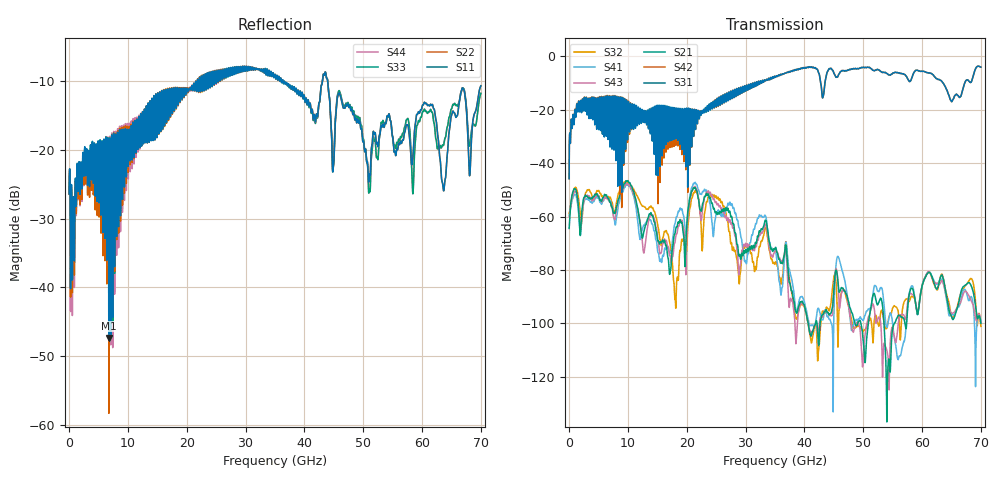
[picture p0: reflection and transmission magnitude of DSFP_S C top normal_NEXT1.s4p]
! AWR Design Environment (8415) Wed Jan 09 11:05:57 2019
! Document = 'DSFP_S'
! nPorts: 4, nXvals: 7001
# HZ S DB R 50
!Freq DBS11 AngS11 DBS12 AngS12 DBS13 AngS13 DBS14 AngS14
!	DBS21 AngS21 DBS22 AngS22 DBS23 AngS23 DBS24 AngS24
!	DBS31 AngS31 DBS32 AngS32 DBS33 AngS33 DBS34 AngS34
!	DBS41 AngS41 DBS42 AngS42 DBS43 AngS43 DBS44 AngS44
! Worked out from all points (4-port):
!   7000 points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, 10 MHz to 70 GHz, reference 50 ohm
!   strongest paths, dB at 10 MHz, 17.51 GHz, 35.01 GHz, 52.51 GHz, 70 GHz:
!     S31: -45.8, -27.6, -7.6, -5.0, -4.0
!     S42: -45.8, -28.8, -7.6, -5.0, -4.0
!     S21: -64.4, -73.0, -72.0, -92.8, -99.9
!     S43: -60.1, -75.6, -73.0, -98.2, -99.8
!     S41: -59.4, -69.8, -72.9, -87.9, -98.9
!     S32: -58.8, -75.9, -77.8, -100.1, -101.1
!   lowest |S11| = -47.4 dB at 6.75 GHz (marker M1), VSWR 1.01, Z = 49.8 + j0.367 ohm
!   |S11| at or under -10 dB: start of sweep to 21.81 GHz; 36.37 GHz to 43.07 GHz (6.701 GHz wide, 16.9 % of centre); 43.96 GHz to end of sweep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
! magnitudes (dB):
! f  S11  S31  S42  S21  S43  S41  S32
! 10 MHz  -26.4  -45.8  -45.8  -64.4  -60.1  -59.4  -58.8
! 1.63 GHz  -23.0  -16.8  -16.7  -57.6  -56.7  -59.0  -53.5
! 6.75 GHz  -47.4  -16.0  -15.8  -53.6  -53.8  -53.4  -52.6
! 17.98 GHz  -12.1  -19.2  -19.8  -66.4  -69.9  -62.8  -90.8
! 21.44 GHz  -10.7  -24.3  -24.2  -49.1  -48.6  -47.2  -50.3
! 28.92 GHz  -8.2  -12.4  -12.4  -74.6  -81.5  -64.2  -85.2
! 70 GHz  -10.7  -4.0  -4.0  -99.9  -99.8  -98.9  -101.1
